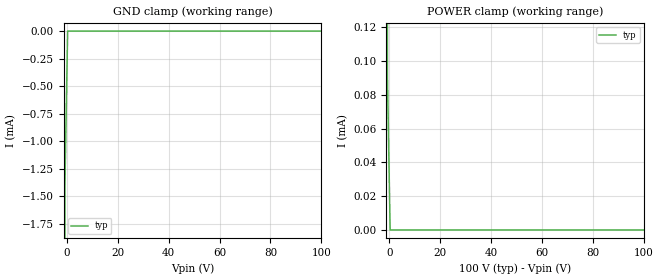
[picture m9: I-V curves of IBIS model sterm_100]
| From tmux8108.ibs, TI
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| sterm_100
[Model]   sterm_100
Model_type   Terminator
|   typ   min   max
C_comp   4.014581e-12   NA   NA
[Voltage Range]   100   NA   NA
[Temperature Range]   27   NA   NA
[Power Clamp Reference]   100   NA   NA
[GND Clamp Reference]   0   NA   NA
[GND Clamp]
|   Voltage   I(typ)   I(min)   I(max)
-5V       -1.144A    NA         NA
-1.818V   -182.5mA   NA         NA
-757.6mV  -1.39mA    NA         NA
303mV     -674.4pA   NA         NA
100V      5.782nA    NA         NA
[POWER Clamp]
|   Voltage   I(typ)   I(min)   I(max)
-5V       744mA      NA         NA
-1.818V   145.4mA    NA         NA
-758mV    90.5uA     NA         NA
303mV     5.779nA    NA         NA
100V      -717.1pA   NA         NA
